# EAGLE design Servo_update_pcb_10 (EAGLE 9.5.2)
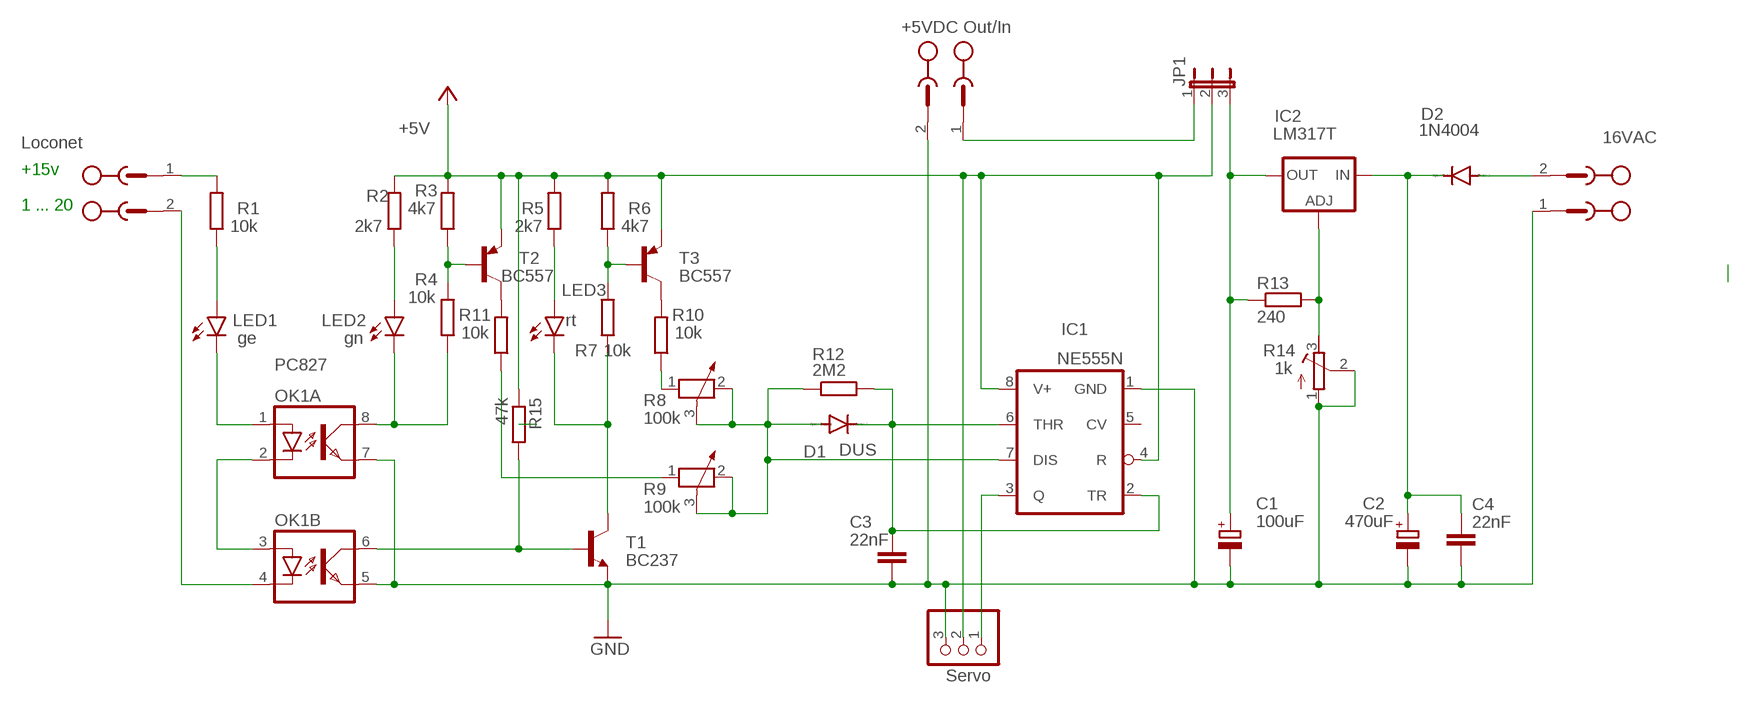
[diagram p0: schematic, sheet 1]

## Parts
1...20  Loconet  MSTBV2  [MSTBV2]
C1  100uF  CPOL-EUE3.5-10  [E3,5-10]
C2  470uF  CPOL-EUE3.5-10  [E3,5-10]
C3  22nF  C-EU050-030X075  [C050-030X075]
C4  22nF  C-EU050-030X075  [C050-030X075]
D1  DUS  1N4148DO35-7  [DO35-7]
D2  1N4004  [DO41-10]
IC1  NE555N  [DIL08]
IC2  LM317T  LM317TS  [317TS]
JP1  JP2E  [JP2]
JP2  Servo  PINHD-1X3  [1X03]
LED1  ge  LED5MM  [LED5MM]
LED2  gn  LED5MM  [LED5MM]
LED3  rt  LED5MM  [LED5MM]
OK1  PC827  [DIL08]
R1  10k  R-EU_0207/10  [0207/10]
R2  2k7  R-EU_0207/10  [0207/10]
R3  4k7  R-EU_0207/10  [0207/10]
R4  10k  R-EU_0207/10  [0207/10]
R5  2k7  R-EU_0207/10  [0207/10]
R6  4k7  R-EU_0207/10  [0207/10]
R7  10k  R-EU_0207/10  [0207/10]
R8  100k  POTENTIOMETER_PT-10  [PT-10]
R9  100k  POTENTIOMETER_PT-10  [PT-10]
R10  10k  R-EU_0207/10  [0207/10]
R11  10k  R-EU_0207/10  [0207/10]
R12  2M2  R-EU_0207/10  [0207/10]
R13  240  R-EU_0207/10  [0207/10]
R14  1k  R-TRIMM64W  [RTRIM64W]
R15  47k  R-EU_0207/10  [0207/10]
T1  BC237  -NPN-TO92  [TO92]
T2  BC557  BC557A-PNP-TO92-EBC  [TO92-EBC]
T3  BC557  BC557A-PNP-TO92-EBC  [TO92-EBC]
X2  16VAC  MSTBV2  [MSTBV2]
X3  +5VDC Out/In  MSTBV2  [MSTBV2]

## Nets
+5V: IC1.4(R) IC1.8(V+) JP1.2 JP2.2 R2.2 R3.2 R5.2 R6.2 R15.1 T2.E T3.E
GND: C1.- C2.- C3.2 C4.2 IC1.1(GND) JP2.3 OK1.5(B:EMIT) OK1.7(A:EMIT) R14.1(A) R14.2(S) T1.1(E) X2.1 X3.2
N$1: LED1.K(C) OK1.1(A:A)
N$2: OK1.2(A:C) OK1.3(B:A)
N$3: 1...20.1 R1.2
N$4: 1...20.2 OK1.4(B:C)
N$5: LED1.A R1.1
N$6: LED2.K(C) OK1.8(A:COL) R4.1
N$7: LED2.A R2.1
N$8: R3.1 R4.2 T2.B
N$9: R10.2 T3.C
N$10: LED3.A R5.1
N$11: R6.1 R7.2 T3.B
N$12: OK1.6(B:COL) R15.2 T1.2(B)
N$13: LED3.K(C) R7.1 T1.3(C)
N$14: R11.2 T2.C
N$15: R8.1 R10.1
N$16: D1.A IC1.7(DIS) R8.2 R8.3 R9.2 R9.3 R12.1
N$17: R9.1 R11.1
N$18: IC2.1(ADJ) R13.2 R14.3(E)
N$19: C3.1 D1.C IC1.2(TR) IC1.6(THR) R12.2
N$20: C2.+ C4.1 D2.C IC2.3(IN)
N$21: D2.A X2.2
N$23: IC1.3(Q) JP2.1
N$24: JP1.1 X3.1
N$27: C1.+ IC2.2(OUT) JP1.3 R13.1
Unconnected: IC1.5(CV)

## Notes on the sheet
- +15v
- 1 ... 20

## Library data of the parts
1...20 X2 X3 = con-phoenix-500:MSTBV2: PHOENIX; OC_FARNELL: unknown; OC_NEWARK: unknown
C1 C2 = rcl:CPOL-EU: POLARIZED CAPACITOR, European symbol; SPICEPREFIX: C
C3 C4 = rcl:C-EU: CAPACITOR, European symbol; SPICEPREFIX: C
D1 = diode:1N4148: DIODE
D2 = diode:1N4004: DIODE
IC1 = linear:*555: TIMER
IC2 = v-reg:LM317TS: VOLTAGE REGULATOR
JP1 = jumper:JP2E: JUMPER
JP2 = pinhead:PINHD-1X3: PIN HEADER
LED1-LED3 = led:LED: LED
OK1 = optocoupler:PC827: SHARP OPTO COUPLER; OC_FARNELL: unknown; OC_NEWARK: unknown
R1-R7 = resistor:R-EU_: RESISTOR, European symbol
R8 R9 = rcl:POTENTIOMETER_: Potentiometer; SPICEMODEL: POT; SPICEPREFIX: X
R10-R13 R15 = rcl:R-EU_: RESISTOR, European symbol; SPICEPREFIX: R
R14 = rcl:R-TRIMM: Trimm resistor; SPICEMODEL: X; SPICEPREFIXL: POT
T1 = transistor:*-NPN-: NPN Transistror BF959 corrected 2008.03.06
T2 T3 = transistor:*-PNP-: PNP Transistror

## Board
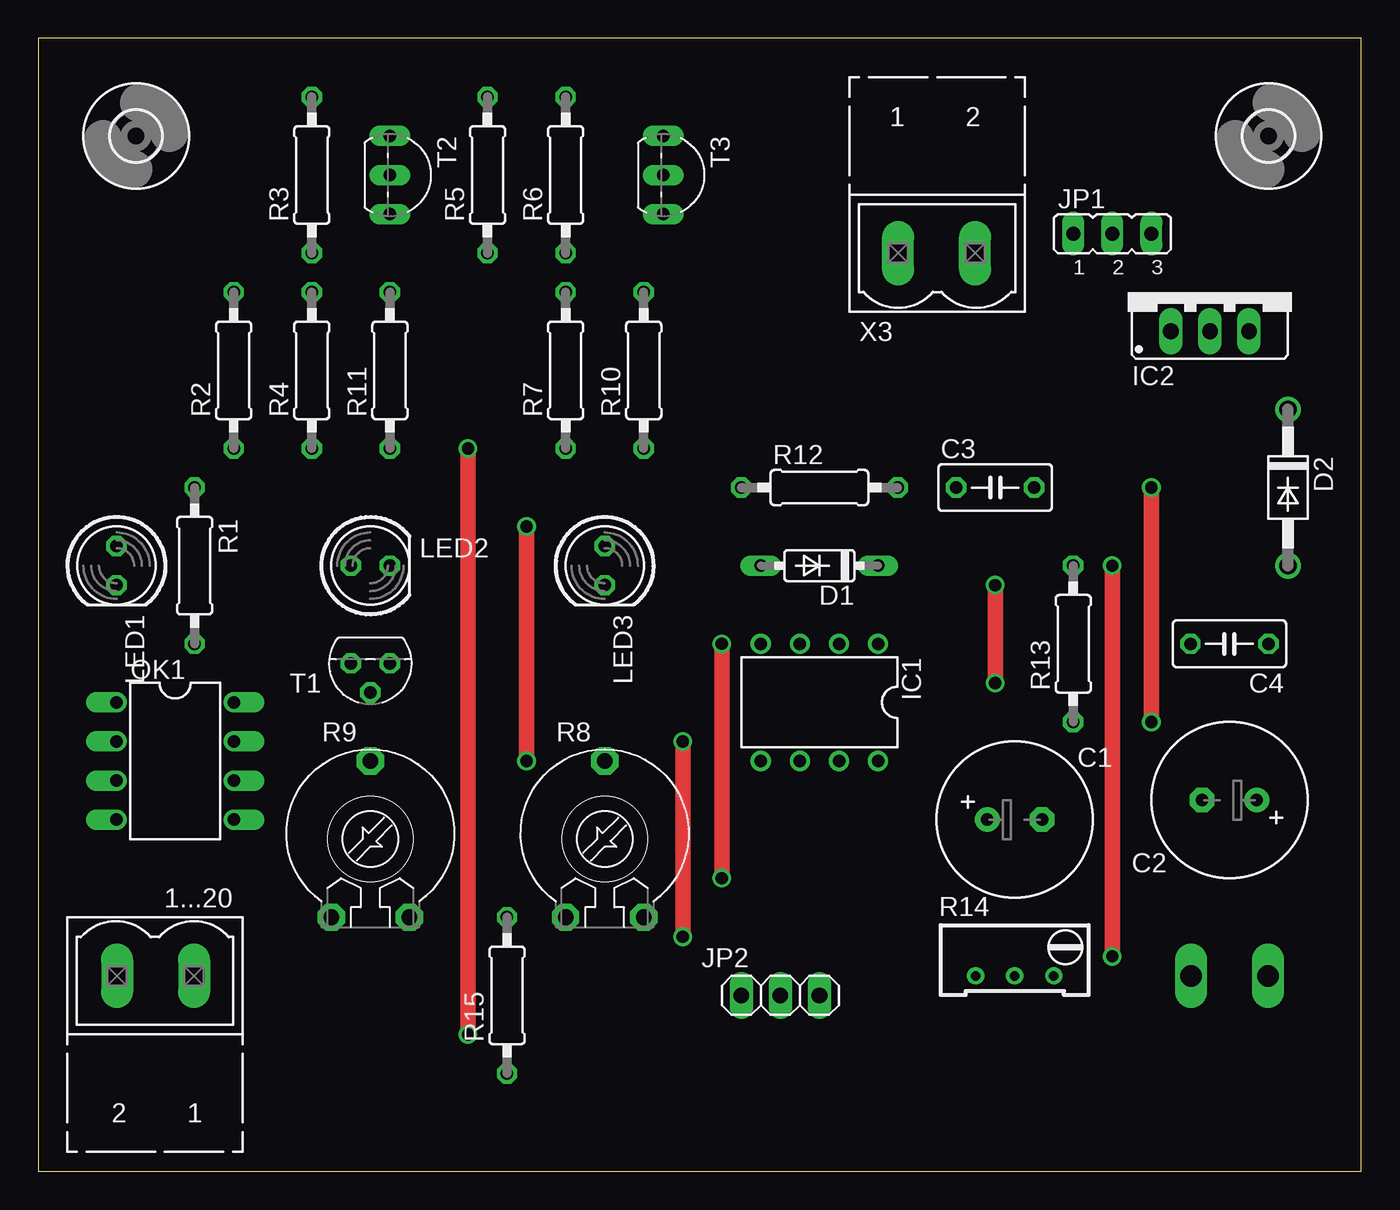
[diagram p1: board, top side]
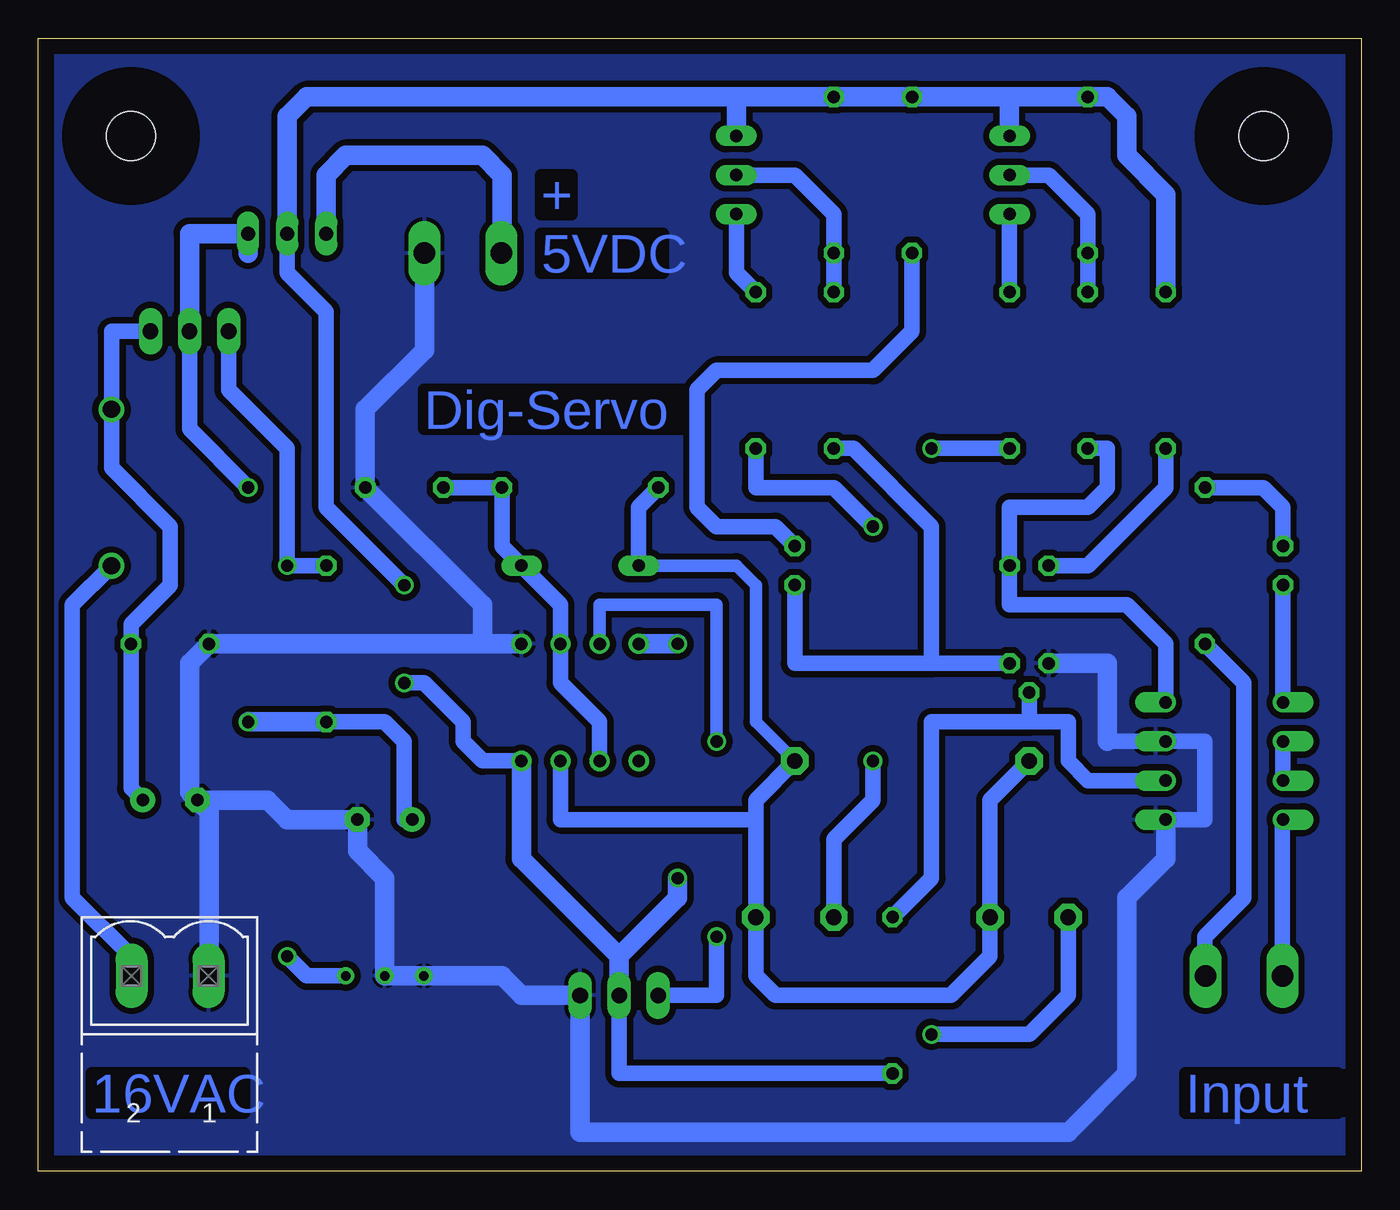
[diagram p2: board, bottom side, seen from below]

Size 86.03 x 73.65 mm. Coordinates in mm from the lower left corner, seen from the top.
Outline: 0,0 86.03,0 86.03,73.65 0,73.65 0,0
Copper layers (1*16): Top 0.035mm / dielectric 1.5mm / Bottom 0.035mm
Design rules "default": minimum track width 6mil, minimum drill 0.35mm, track to track 6mil, track to pad 6mil, pad to pad 6mil, via to via 6mil, smd to smd 6mil, copper to edge 40mil, drill to drill 6mil, minimum pad ring 10mil, minimum via ring 8mil, stop-mask expansion 4mil, vias tented up to drill 0mil, thermal gap 10mil

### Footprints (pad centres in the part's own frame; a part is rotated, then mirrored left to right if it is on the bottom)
MSTBV2 = drill 1.397 long: 1 -2.5,0; 2 2.5,0
E3,5-10 = drill 0.813 pad 1.6: + -1.778,0 | drill 0.813 pad 1.6 octagon: - 1.778,0
C050-030X075 = drill 0.813 octagon: 1 -2.54,0; 2 2.54,0
DO35-7 = drill 0.813 long: A 3.81,0; C -3.81,0
DO41-10 = drill 1.118: A 5.08,0; C -5.08,0
DIL08 = drill 0.813 pad 1.27: 1 -3.81,-3.81; 2 -1.27,-3.81; 3 1.27,-3.81; 4 3.81,-3.81; 5 3.81,3.81; 6 1.27,3.81; 7 -1.27,3.81; 8 -3.81,3.81
317TS = drill 1.016 long: 1 -2.54,-2.54; 2 0,-2.54; 3 2.54,-2.54
JP2 = drill 0.914 long: 1 -2.54,0; 2 0,0; 3 2.54,0
1X03 = drill 1.016 long: 1 -2.54,0; 2 0,0; 3 2.54,0
LED5MM = drill 0.813 octagon: A -1.27,0; K 1.27,0
DIL08' = drill 0.813 offset: 1 -3.81,-3.81; 2 -1.27,-3.81; 3 1.27,-3.81; 4 3.81,-3.81; 5 3.81,3.81; 6 1.27,3.81; 7 -1.27,3.81; 8 -3.81,3.81
0207/10 = drill 0.813 octagon: 1 -5.08,0; 2 5.08,0
PT-10 = drill 1.016 pad 1.778 octagon: 1 -2.54,-5.08; 2 2.54,-5.08; 3 0,5.08
RTRIM64W = drill 0.61: 1 1.27,-2.54; 2 1.27,0; 3 1.27,2.54
TO92 = drill 0.813 octagon: 1 1.27,0; 2 0,1.905; 3 -1.27,0
TO92-EBC = drill 0.813 long: B 0,-1.27; C 2.54,-1.27; E -2.54,-1.27
3,2 = hole 3.2: 0,0

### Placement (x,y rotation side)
1...20  7.62,12.7 180 top
C1  63.5,22.86 0 top
C2  77.47,24.13 180 top
C3  62.23,44.45 0 top
C4  77.47,34.29 180 top
D1  50.8,39.37 180 top
D2  81.28,44.45 270 top
IC1  50.8,30.48 180 top
IC2  76.2,57.15 0 top
JP1  69.85,60.96 0 top
JP2  48.26,11.43 0 top
LED1  5.08,39.37 270 top
LED2  21.59,39.37 0 top
LED3  36.83,39.37 270 top
OK1  PC827  [DIL08']  8.89,26.67 270 top
R1  10.16,39.37 270 top
R2  12.7,52.07 90 top
R3  17.78,64.77 90 top
R4  17.78,52.07 90 top
R5  29.21,64.77 90 top
R6  34.29,64.77 90 top
R7  34.29,52.07 90 top
R8  36.83,21.59 0 top
R9  21.59,21.59 0 top
R10  39.37,52.07 90 top
R11  22.86,52.07 90 top
R12  50.8,44.45 0 top
R13  67.31,34.29 90 top
R14  63.5,13.97 270 top
R15  30.48,11.43 90 top
T1  21.59,33.02 180 top
T2  24.13,64.77 270 top
T3  41.91,64.77 270 top
U$1  [3,2]  80.01,67.31 0 top
U$2  [3,2]  6.35,67.31 0 top
X2  77.47,12.7 180 bottom
X3  58.42,59.69 0 top

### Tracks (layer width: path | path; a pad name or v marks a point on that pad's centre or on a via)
+5V  (via drill 0.35, 0.8)
  Top 1.016: v44.45,34.29 v44.45,19.05 | v62.23,31.75 v62.23,38.1
  Bottom 1.016: JP2.2 48.26,6.35 R15.1 | IC1.8 57.15,26.67 58.42,27.94 58.42,29.21 60.96,31.75 v62.23,31.75 | v62.23,38.1 67.31,43.18 67.31,55.88 69.85,58.42 JP1.2
  Bottom 1.27: 22.86,69.85 R3.2 16.51,69.85 15.24,68.58 15.24,66.04 12.7,63.5 R2.2 | T2.E 22.86,69.85 | 22.86,69.85 R5.2 R6.2 40.64,69.85 | 40.64,69.85 T3.E | 48.26,13.97 54.61,20.32 IC1.8 | 48.26,13.97 JP2.2 | IC1.4 v44.45,34.29 | v44.45,19.05 44.45,17.78 48.26,13.97 | 40.64,69.85 68.58,69.85 69.85,68.58 JP1.2
GND
  Bottom 1.016: 16.51,27.94 OK1.7 10.16,27.94 10.16,22.86 OK1.5 | 74.93,12.74 X2.1
  Bottom 1.27: 16.51,27.94 16.51,33.02 T1.1 | IC1.1 57.15,34.29 | 57.15,34.29 57.15,36.83 C3.2 64.77,49.53 60.92,53.38 X3.2 | 57.15,34.29 C4.2 76.2,33.02 76.2,24.64 C2.- | C2.- 71.12,24.13 69.85,22.86 C1.- 65.28,20.83 63.5,19.05 R14.2 R14.1 55.88,12.7 54.61,11.43 JP2.3 50.8,2.54 19.05,2.54 15.24,6.35 15.24,17.78 12.7,20.32 OK1.5 | C2.- 74.93,23.37 74.93,12.74
  pour Bottom (isolate 0.406): 0,73.66 86.36,73.66 86.36,0 0,0
N$1
  Bottom 1.016: LED1.K OK1.1
N$2
  Bottom 1.016: OK1.2 OK1.3
N$3
  Bottom 1.016: 1...20.1 10.16,12.74 10.16,15.24 7.62,17.78 7.62,31.75 R1.2
N$4
  Bottom 1.016: 1...20.2 5.12,22.82 OK1.4
N$5
  Bottom 1.016: LED1.A 5.08,43.18 6.35,44.45 R1.1
N$6
  Bottom 1.016: R4.1 16.51,46.99 16.51,44.45 17.78,43.18 22.86,43.18 LED2.K 22.86,36.83 15.24,36.83 12.7,34.29 OK1.8
N$7
  Bottom 1.016: R2.1 12.7,44.45 17.78,39.37 LED2.A
N$8
  Bottom 1.016: R4.2 R3.1 17.78,62.23 20.32,64.77 T2.B
N$9
  Bottom 1.016: T3.C 40.64,58.42 R10.2
N$10
  Bottom 1.016: R5.1 29.21,54.61 31.75,52.07 41.91,52.07 43.18,50.8 43.18,43.18 41.91,41.91 38.1,41.91 LED3.A
N$11
  Bottom 1.016: R7.2 R6.1 34.29,62.23 36.83,64.77 T3.B
N$12
  Bottom 1.016: OK1.6 17.78,25.4 19.05,26.67 19.05,29.21 21.59,29.21 | 21.59,29.21 T1.2 | R15.2 27.94,19.05 27.94,29.21 21.59,29.21
N$13
  Bottom 1.016: T1.3 27.94,33.02 | LED3.K 36.83,33.02 27.94,33.02 | R7.1 33.02,46.99 27.94,41.91 27.94,33.02
N$14
  Bottom 1.016: T2.C R11.2
N$15  (via drill 0.8)
  Top 1.016: v31.75,41.91 v31.75,26.67
  Bottom 1.016: v31.75,26.67 31.75,24.13 34.29,21.59 R8.1 | v31.75,41.91 34.29,44.45 39.37,44.45 R10.1
N$16
  Bottom 0.813: D1.A 40.64,39.37 39.37,38.1 39.37,29.21 R8.3
  Bottom 1.016: R9.3 24.13,24.13 R9.2 24.13,13.97 26.67,11.43 38.1,11.43 39.37,12.7 R8.2 39.37,22.86 | R8.3 39.37,24.13 39.37,22.86 | IC1.7 52.07,22.86 39.37,22.86 | R12.1 46.99,43.18 D1.A
N$17  (via drill 0.8)
  Top 1.016: v27.94,46.99 v27.94,8.89
  Bottom 1.016: R11.1 v27.94,46.99 | R9.1 19.05,11.43 21.59,8.89 v27.94,8.89
N$18  (via drill 0.8)
  Top 1.016: v69.85,39.37 v69.85,13.97
  Bottom 1.016: v69.85,13.97 68.58,12.7 R14.3 | IC2.1 73.66,50.8 69.85,46.99 v69.85,39.37 R13.2
N$19
  Bottom 1.016: C3.1 R12.2 55.88,40.64 D1.C 52.07,36.83 IC1.2 52.07,31.75 49.53,29.21 IC1.6
N$20
  Bottom 1.016: C2.+ 80.01,24.89 C4.1 80.01,35.56 77.47,38.1 77.47,41.91 81.28,45.72 D2.C 81.28,54.61 IC2.3
N$21
  Bottom 1.016: D2.A 83.82,36.83 83.82,17.78 80.01,13.97 80.01,11.43 79.97,11.47 X2.2
N$23  (via drill 0.8)
  Top 1.016: v41.91,27.94 v41.91,15.24
  Bottom 0.508: 41.93,36.83 41.91,36.81
  Bottom 0.813: IC1.3 49.53,36.83 41.93,36.83 | 41.91,36.81 v41.91,27.94
  Bottom 1.016: v41.91,15.24 41.91,11.43 JP2.1
N$24
  Bottom 1.27: X3.1 55.88,59.73 55.88,64.77 57.15,66.04 66.04,66.04 67.31,64.77 JP1.1
N$27  (via drill 0.8)
  Top 1.016: v72.39,44.45 v72.39,29.21
  Bottom 1.016: R13.1 63.5,29.21 62.23,27.94 62.23,22.86 C1.+ | IC2.2 76.2,48.26 v72.39,44.45
  Bottom 1.27: v72.39,29.21 R13.1 | IC2.2 76.2,60.96 JP1.3 72.39,59.69

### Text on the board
Bottom: + | 5VDC | Dig-Servo | Input | 16VAC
